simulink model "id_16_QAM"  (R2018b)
settings: Solver=VariableStepAuto  StartTime=0.0  StopTime=inf  RelTol=1e-3
libraries: commfilt2 x2, commdigbbndam3 x2, commchan3 x1, commrandsrc3 x1, commsink2 x1, commutil2 x1

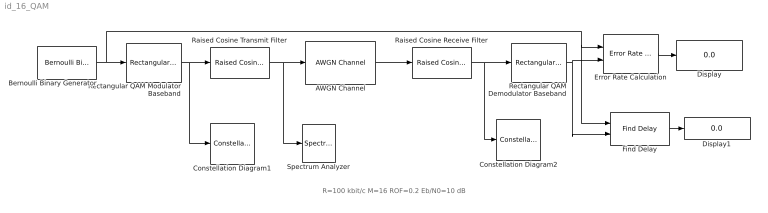
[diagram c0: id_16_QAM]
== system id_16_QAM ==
  note: R=100 kbit/c M=16 ROF=0.2 Eb/N0=10 dB
  AWGN Channel : commchan3/AWGN Channel  InputProcessing=Columns as channels (frame based)  seed=67  noiseMode="Signal to noise ratio  (Eb/No)"  EbNodB=10  EsNodB=10  SNRdB=10  bitsPerSym=4  Ps=1/8  Tsym=1/200e3  variance=1
  Bernoulli Binary Generator : commrandsrc3/Bernoulli Binary Generator  ProbabilityOfZero=0.5  SeedSource=Auto  Seed=0  SampleTime=1/800e3  SamplesPerFrame=200  OutputDataType=double  SimulateUsing=Interpreted execution
  Constellation Diagram1 : ConstellationDiagram
  Constellation Diagram2 : ConstellationDiagram
  Display : Display
  Display1 : Display
  Error Rate Calculation : commsink2/Error Rate Calculation  N=40  st_delay=0  cp_mode=Entire frame  subframe=[]  PMode=Port  WsName=ErrorVec  RsMode2=off  stop=off  numErr=100  maxBits=1e6
  Find Delay : commutil2/Find Delay  corrLength=400  chgSigOP=off  stopUpdate=off  numConstDelay=3
  Raised Cosine Receive Filter : commfilt2/Raised Cosine Receive Filter  filtType=Square root  R=0.2  filtSpan=10  N=8  downFactor=8  downOffset=0  filterGain=1  InputProcessing=Columns as channels (frame based)  RateOptions=Enforce single-rate processing  framing=Mute  checkCoeff=off  variableName=rcRxFilt  currentFiltSpan=10  D=5  inputOffset=0  sampMode=Mute  saveAsFlag=0  rateMode=Downsampling  checkGain=Normalized  launchFVT=on  roundingMode=Floor  overflowMode=off  coeffDataTypeStr=Inherit: Same word length as input  coeffMin=[]  coeffMax=[]  coeffLastDataTypeStr=Inherit: Same word length as input  accumDataTypeStr=Inherit: Same as product output  accumLastDataTypeStr=Inherit: Same as product output  outputDataTypeStr=Inherit: Same as accumulator  outputMin=[]  outputMax=[]  outputLastDataTypeStr=Inherit: Same as accumulator
  Raised Cosine Transmit Filter : commfilt2/Raised Cosine Transmit Filter  filtType=Square root  R=0.2  filtSpan=10  N=8  filterGain=1  InputProcessing=Columns as channels (frame based)  RateOptions=Enforce single-rate processing  framing=Mute  checkCoeff=off  variableName=rcTxFilt  checkGain=Normalized  sampMode=Mute  saveAsFlag=0  currentFiltSpan=10  D=(10)/2  launchFVT=on  roundingMode=Floor  overflowMode=off  coeffDataTypeStr=Inherit: Same word length as input  coeffMin=[]  coeffMax=[]  coeffLastDataTypeStr=Inherit: Same word length as input  outputDataTypeStr=Inherit: Same as accumulator  outputMin=[]  outputMax=[]  outputLastDataTypeStr=Inherit: Same as accumulator
  Rectangular QAM Demodulator Baseband : commdigbbndam3/Rectangular QAM Demodulator Baseband  M=16  OutType=Bit  DecType=Hard decision  VarSource=Dialog  Variance=1  Dec=Gray  Mapping=[0:15]  PowType=Average Power  MinDist=2  AvgPow=1  PeakPow=1  Ph=0  outDtype1=Inherit via internal rule  outDtype2=Inherit via internal rule  derotateFactorWordLen=16  derotateFactorDataTypeStr=Inherit: Same word length as input  derotateFactorLastDataTypeStr=Inherit: Same word length as input  denormFactorWordLen=16  denormFactorDataTypeStr=Inherit: Same word length as input  denormFactorLastDataTypeStr=Inherit: Same word length as input  prodOutWordLen=32  prodOutOverflowMode=Wrap  prodOutRoundingMode=Floor  prodOutOvFlMode=off  prodOutOvFlModeLastStrValue=off  sumWordLen=32
  Rectangular QAM Modulator Baseband : commdigbbndam3/Rectangular QAM Modulator Baseband  M=16  InType=Bit  Enc=Gray  Mapping=[0:15]  PowType=Average Power  MinDist=2  AvgPow=1  PeakPow=1  Ph=0  outDtype=double  outWordLen=16  outUDDataType=sfix(16)  outFracLenMode=Best precision  outFracLen=15  outDataTypeStr=double  outLastDataTypeStr=double
  Spectrum Analyzer : SpectrumAnalyzer
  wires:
  Bernoulli Binary Generator/1 -> Rectangular QAM Modulator Baseband/1, Find Delay/1, Error Rate Calculation/1
  Rectangular QAM Modulator Baseband/1 -> Constellation Diagram1/1, Raised Cosine Transmit Filter/1
  Raised Cosine Transmit Filter/1 -> AWGN Channel/1, Spectrum Analyzer/1
  AWGN Channel/1 -> Raised Cosine Receive Filter/1
  Raised Cosine Receive Filter/1 -> Rectangular QAM Demodulator Baseband/1, Constellation Diagram2/1
  Rectangular QAM Demodulator Baseband/1 -> Find Delay/2, Error Rate Calculation/2
  Find Delay/1 -> Display1/1
  Error Rate Calculation/1 -> Display/1
